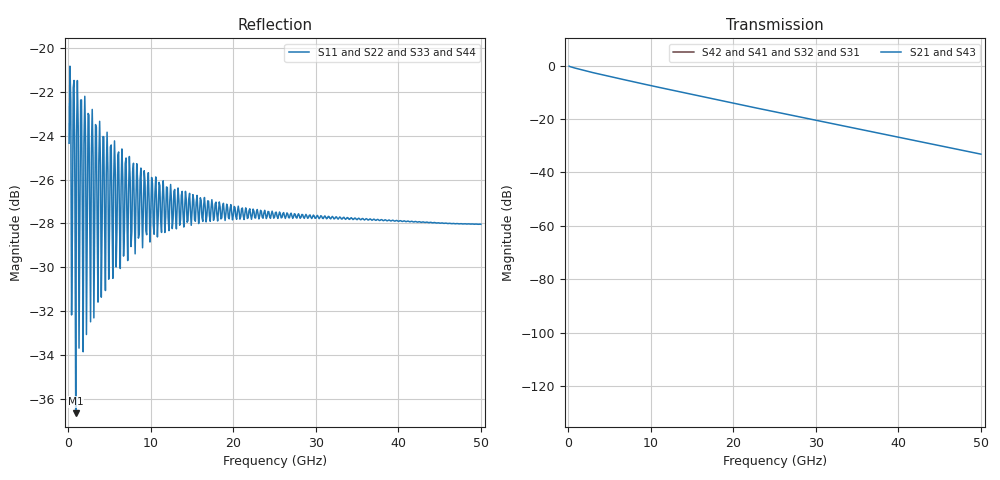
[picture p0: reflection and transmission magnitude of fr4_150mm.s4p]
! Touchstone Ver. 1.0
! Number of ports is 4
! port1 ->  port2
! port3 ->  port4
# Hz	S	RI	R	50.000000
! SCATTERING PARAMETERS  :
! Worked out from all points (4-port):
!   500 points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, 100 MHz to 50 GHz, reference 50 ohm
!   strongest paths, dB at 100 MHz, 12.6 GHz, 25.1 GHz, 37.6 GHz, 50 GHz:
!     S21: -0.2, -9.2, -17.4, -25.3, -33.2
!     S43: -0.2, -9.2, -17.4, -25.3, -33.2
!     S42: -, -, -, -, -
!     S41: -, -, -, -, -
!     S32: -, -, -, -, -
!     S31: -, -, -, -, -
!   lowest |S11| = -36.7 dB at 900 MHz (marker M1), VSWR 1.03, Z = 48.9 - j0.918 ohm
!   |S11| at or under -10 dB: start of sweep to end of sweep
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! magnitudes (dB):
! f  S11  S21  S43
! 100 MHz  -24.3  -0.2  -0.2
! 300 MHz  -22.4  -0.5  -0.5
! 900 MHz  -36.7  -1.0  -1.0
! 1.1 GHz  -21.5  -1.2  -1.2
! 1.3 GHz  -33.7  -1.3  -1.3
! 2 GHz  -22.2  -1.9  -1.9
! 50 GHz  -28.0  -33.2  -33.2
